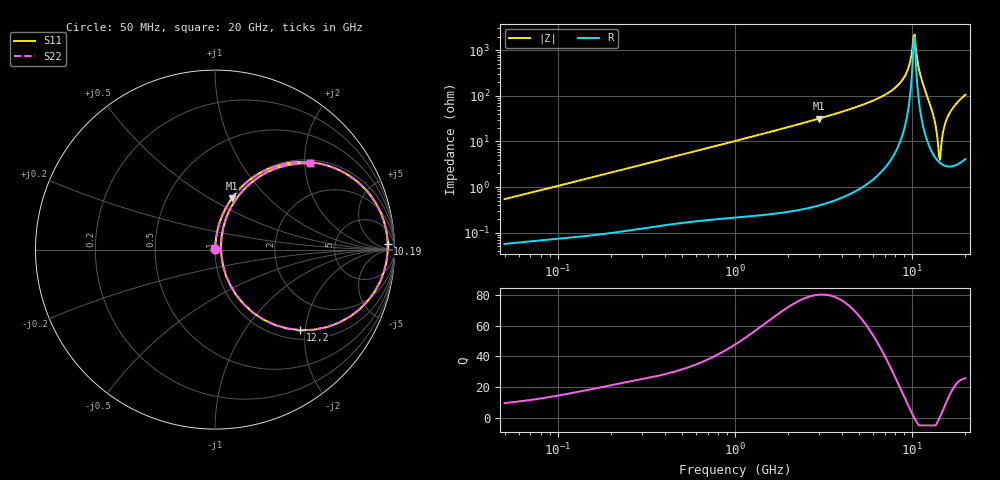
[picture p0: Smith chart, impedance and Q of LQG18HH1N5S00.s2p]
!Murata Part Number: LQG18HH1N5S00
!These Parameters are Measured in Series Mode Connection
!  o--[Z]--o
!Port1  Port2
!  o-------o
!Freq. Start=50[MHz] Stop=20[GHz], 401[Steps]
# Hz S RI R 50
!Freq.(Hz) S11(Real) S11(Imag) S21(Real) S21(Imag) S12(Real) S12(Imag) S22(Real) S22(Imag)
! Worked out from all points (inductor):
!   401 points, 50 MHz to 20 GHz, reference 50 ohm
!   read as one part in series: L = 1.71 nH near 51.52 MHz
!   highest Q = 80.3 at 2.985 GHz (marker M1), where L = 1.7 nH
!   self-resonance near 10.19 GHz
!   S11 on the Smith chart (normalised r, x): 50 MHz: 1.00, +0.01; 10.19 GHz: 32, +26; 12.2 GHz: 1.20, -1.89; 20 GHz: 1.08, +2.12
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5e7  0.000596 0.00541  0.9994 -0.00541  0.9994 -0.00541  0.000596 0.00541
1.364002e8  0.00103 0.0143  0.999 -0.0143  0.999 -0.0143  0.00103 0.0143
3.721004e8  0.00286 0.0383  0.9971 -0.0383  0.9971 -0.0383  0.00286 0.0383
1e9  0.0124 0.1007  0.9876 -0.1007  0.9876 -0.1007  0.0124 0.1007
2.728004e9  0.0794 0.2642  0.9206 -0.2642  0.9206 -0.2642  0.0794 0.2642
2.98453e9  0.0947 0.2866  0.9053 -0.2866  0.9053 -0.2866  0.0947 0.2866
5.041459e9  0.2685 0.4357  0.7315 -0.4357  0.7315 -0.4357  0.2685 0.4357
7.442007e9  0.5915 0.4772  0.4085 -0.4772  0.4085 -0.4772  0.5915 0.4772
9.178299e9  0.873 0.2932  0.127 -0.2932  0.127 -0.2932  0.873 0.2932
9.600142e9  0.926 0.1994  0.074 -0.1994  0.074 -0.1994  0.926 0.1994
1.019291e10  0.9627 0.0301  0.0373 -0.0301  0.0373 -0.0301  0.9627 0.0301
1.050288e10  0.9544 -0.0719  0.0456 0.0719  0.0456 0.0719  0.9544 -0.0719
1.098561e10  0.8901 -0.2334  0.1099 0.2334  0.1099 0.2334  0.8901 -0.2334
1.131968e10  0.8059 -0.3323  0.1941 0.3323  0.1941 0.3323  0.8059 -0.3323
1.220001e10  0.4763 -0.449  0.5237 0.449  0.5237 0.449  0.4763 -0.449
1.314879e10  0.1601 -0.3043  0.8399 0.3043  0.8399 0.3043  0.1601 -0.3043
1.396067e10  0.0447 -0.0883  0.9553 0.0883  0.9553 0.0883  0.0447 -0.0883
1.438523e10  0.0331 0.0192  0.9669 -0.0192  0.9669 -0.0192  0.0331 0.0192
1.460232e10  0.0364 0.0694  0.9636 -0.0694  0.9636 -0.0694  0.0364 0.0694
1.527346e10  0.0725 0.2018  0.9275 -0.2018  0.9275 -0.2018  0.0725 0.2018
1.621653e10  0.1587 0.3323  0.8413 -0.3323  0.8413 -0.3323  0.1587 0.3323
2e10  0.5277 0.4801  0.4723 -0.4801  0.4723 -0.4801  0.5277 0.4801
